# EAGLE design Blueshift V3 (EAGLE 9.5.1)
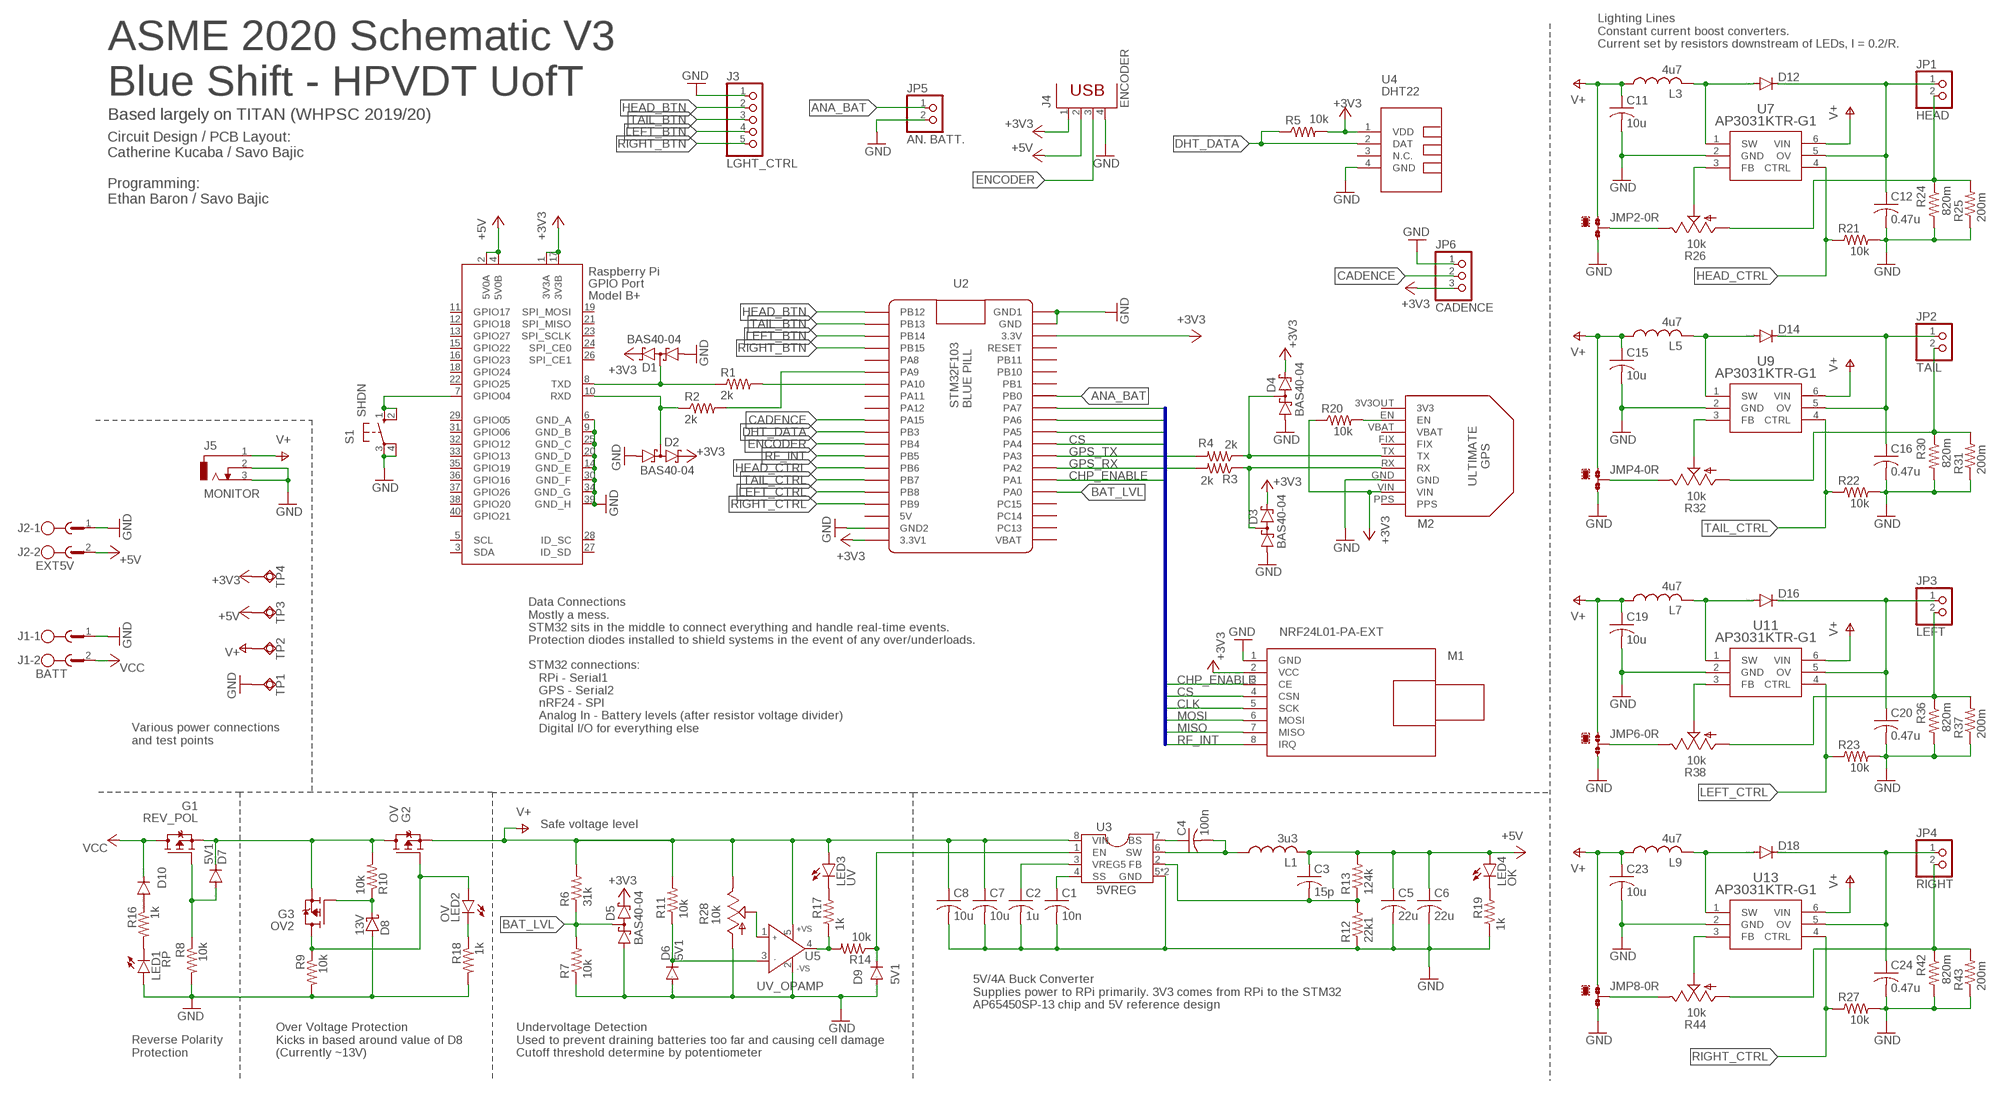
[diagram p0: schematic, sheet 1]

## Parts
C1  10n  C-USC0402  [C0402]
C2  1u  C-USC0402  [C0402]
C3  15p  C-USC0402  [C0402]
C4  100n  C-USC0402  [C0402]
C5  22u  C-USC0805  [C0805]
C6  22u  C-USC0805  [C0805]
C7  10u  C-USC0805  [C0805]
C8  10u  C-USC0805  [C0805]
C11  10u  C-USC1206K  [C1206K]
C12  0.47u  C-USC1206K  [C1206K]
C15  10u  C-USC1206K  [C1206K]
C16  0.47u  C-USC1206K  [C1206K]
C19  10u  C-USC1206K  [C1206K]
C20  0.47u  C-USC1206K  [C1206K]
C23  10u  C-USC1206K  [C1206K]
C24  0.47u  C-USC1206K  [C1206K]
D1  BAS40-04  [SOT23]
D2  BAS40-04  [SOT23]
D3  BAS40-04  [SOT23]
D4  BAS40-04  [SOT23]
D5  BAS40-04  [SOT23]
D6  5V1  DIODE-SOD323-R  [SOD323-R]
D7  5V1  DIODE-SOD323-R  [SOD323-R]
D8  13V  BAS70  [SOT23]
D9  5V1  DIODE-SOD323-R  [SOD323-R]
D10  DIODE-SOD80C  [SOD80C]
D12  DIODE-DO-214AC  [DO-214AC]
D14  DIODE-DO-214AC  [DO-214AC]
D16  DIODE-DO-214AC  [DO-214AC]
D18  DIODE-DO-214AC  [DO-214AC]
G1  REV_POL  SI3493DDV-T1-GE3  [TSOP-6]
G2  OV  SI3493DDV-T1-GE3  [TSOP-6]
G3  OV2  SI3493DDV-T1-GE3  [TSOP-6]
J1  BATT  MST2V  [MSTBV2]
J2  EXT5V  MST2V  [MSTBV2]
J3  LGHT_CTRL  PINHD-1X5  [1X05]
J4  ENCODER  PN87520  [PN87520]
J5  MONITOR  DCJ0303  [DCJ0303]
JMP2  0R-JUMPA  [A0R-JMP]
JMP4  0R-JUMPA  [A0R-JMP]
JMP6  0R-JUMPA  [A0R-JMP]
JMP8  0R-JUMPA  [A0R-JMP]
JP1  HEAD  PINHD-1X2  [1X02]
JP2  TAIL  PINHD-1X2  [1X02]
JP3  LEFT  PINHD-1X2  [1X02]
JP4  RIGHT  PINHD-1X2  [1X02]
JP5  AN. BATT.  PINHD-1X2  [1X02]
JP6  CADENCE  PINHD-1X3  [1X03]
L1  3u3  SDES064T-3R3MS  [SDES064T]
L3  4u7  NR6028NR6028  [INDDFN600X600X280-2N]
L5  4u7  NR6028NR6028  [INDDFN600X600X280-2N]
L7  4u7  NR6028NR6028  [INDDFN600X600X280-2N]
L9  4u7  NR6028NR6028  [INDDFN600X600X280-2N]
LED1  RP  LEDSML0805  [SML0805]
LED2  OV  LEDSML0805  [SML0805]
LED3  UV  LEDSML0805  [SML0805]
LED4  OK  LEDSML0805  [SML0805]
M1  NRF24L01-PA-EXT  WIRELESS-NRF24L01-PA-EXT  [WIRELESS-NRF24L01-PA-EXT]
M2  ULTIMATE-GPS  [ULTIMATE_GPS]
R1  2k  R-US_R0402  [R0402]
R2  2k  R-US_R0402  [R0402]
R3  2k  R-US_R0402  [R0402]
R4  2k  R-US_R0402  [R0402]
R5  10k  R-US_R0402  [R0402]
R6  31k  R-US_R0402  [R0402]
R7  10k  R-US_R0402  [R0402]
R8  10k  R-US_R0402  [R0402]
R9  10k  R-US_R0402  [R0402]
R10  10k  R-US_R0402  [R0402]
R11  10k  R-US_R0402  [R0402]
R12  22k1  R-US_R0402  [R0402]
R13  124k  R-US_R0402  [R0402]
R14  10k  R-US_R0402  [R0402]
R16  1k  R-US_R0402  [R0402]
R17  1k  R-US_R0402  [R0402]
R18  1k  R-US_R0402  [R0402]
R19  1k  R-US_R0402  [R0402]
R20  10k  R-US_R0402  [R0402]
R21  10k  R-US_R0402  [R0402]
R22  10k  R-US_R0402  [R0402]
R23  10k  R-US_R0402  [R0402]
R24  820m  R-US_R0603  [R0603]
R25  200m  R-US_R0805  [R0805]
R26  10k  TRIM_US-RJ9W  [RJ9W]
R27  10k  R-US_R0402  [R0402]
R28  10k  TRIM_US-RJ9W  [RJ9W]
R30  820m  R-US_R0603  [R0603]
R31  200m  R-US_R0805  [R0805]
R32  10k  TRIM_US-RJ9W  [RJ9W]
R36  820m  R-US_R0603  [R0603]
R37  200m  R-US_R0805  [R0805]
R38  10k  TRIM_US-RJ9W  [RJ9W]
R42  820m  R-US_R0603  [R0603]
R43  200m  R-US_R0805  [R0805]
R44  10k  TRIM_US-RJ9W  [RJ9W]
S1  SHDN  10-XX  [B3F-10XX]
TP1  TPSQTP20SQ  [TP20SQ]
TP2  TPSQTP20R  [TP20R]
TP3  TPSQTP20R  [TP20R]
TP4  TPSQTP20R  [TP20R]
U1  RASPI_HAT  [RASPI_BOARD_B+HAT_CF]
U2  BLUEPILL  BLUE_PILL  [BLUE_PILL]
U3  5VREG  AP65450SP-13  [SO-8EP]
U4  DHT22  TEMP-HUM-SENSOR-DHT22  [TEMP-HUM-SENSOR-DHT22]
U5  UV_OPAMP  TA75S558F,LF  [SOT-753]
U7  AP3031KTR-G1  [SOT23-6]
U9  AP3031KTR-G1  [SOT23-6]
U11  AP3031KTR-G1  [SOT23-6]
U13  AP3031KTR-G1  [SOT23-6]

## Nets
5V_FB: C3.2 R12.2 R13.1 U3.2(FB)
+3V3: D1.2(C2) D2.2(C2) D3.2(C2) D4.2(C2) D5.2(C2) J4.1 JP6.3 M1.2(VCC) M2.VIN R5.2 R20.1 TP4.TP U1.1(3V3A) U1.17(3V3B) U2.P$20(3.3V1) U2.P$23(3.3V) U4.1(VDD)
+5V: C3.1 C5.1 C6.1 J2.2 J4.2 L1.2 LED4.A R13.2 TP3.TP U1.2(5V0A) U1.4(5V0B)
ANA_BAT: JP5.1 U2.P$28(PB0)
BAT_LVL: D5.3(C1A2) R6.1 R7.2 U2.P$36(PA0)
CADENCE: JP6.2 U2.P$10(PA15)
CHP_ENABLE: M1.3(CE) U2.P$35(PA1)
CLK: M1.5(SCK) U2.P$31(PA5)
CS: M1.4(CSN) U2.P$32(PA4)
DHT_DATA: R5.1 U2.P$11(PB3) U4.2(DAT)
ENCODER: J4.3 U2.P$12(PB4)
GND: C1.2 C2.2 C5.2 C6.2 C7.2 C8.2 C11.2 C12.2 C15.2 C16.2 C19.2 C20.2 C23.2 C24.2 D1.1(A1) D2.1(A1) D3.1(A1) D4.1(A1) D5.1(A1) D6.A D8.1(A) D9.A J1.1 J2.1 J3.1 J4.4 J5.2 J5.3 JMP2.3 JMP4.3 JMP6.3 JMP8.3 JP5.2 JP6.1 LED1.A M1.1(GND) M2.GND R7.1 R8.2 R9.2 R12.1 R18.2 R19.1 R21.2 R22.2 R23.2 R24.2 R25.1 R27.2 R28.A R30.2 R31.1 R36.2 R37.1 R42.2 R43.1 S1.3(P) S1.4(P1) TP1.TP U1.6(GND_A) U1.9(GND_B) U1.14(GND_E) U1.20(GND_D) U1.25(GND_C) U1.30(GND_F) U1.34(GND_G) U1.39(GND_H) U2.P$19(GND2) U2.P$21(GND1) U2.P$22(GND) U3.5(GND) U3.TP(GND) U4.4(GND) U5.2(-VS) U7.2(GND) U9.2(GND) U11.2(GND) U13.2(GND)
GPS_RX: R3.2 U2.P$34(PA2)
GPS_TX: R4.2 U2.P$33(PA3)
HEAD_BTN: J3.2 U2.P$1(PB12)
HEAD_CTRL: R21.1 U2.P$14(PB6) U7.4(CTRL)
LEFT_BTN: J3.4 U2.P$3(PB14)
LEFT_CTRL: R23.1 U2.P$16(PB8) U11.4(CTRL)
MISO: M1.7(MISO) U2.P$30(PA6)
MOSI: M1.6(MOSI) U2.P$29(PA7)
N$1: R1.2 U2.P$7(PA10)
N$2: R2.2 U2.P$6(PA9)
N$3: D1.3(C1A2) R1.1 U1.8(TXD)
N$4: D2.3(C1A2) R2.1 U1.10(RXD)
N$5: D3.3(C1A2) M2.RX R3.1
N$6: S1.1(S) S1.2(S1) U1.7(GPIO04)
N$7: D8.3(C) G3.3(G) R10.1
N$8: D7.A G1.3(G) R8.1
N$9: D4.3(C1A2) M2.TX R4.1
N$10: G2.3(G) G3.1(D) G3.2(D) G3.5(D) G3.6(D) LED2.A R9.1
N$11: LED3.C R17.2
N$12: C1.1 U3.4(SS)
N$13: D6.C R11.1 U5.3(IN-)
N$14: C4.2 L1.1 U3.6(SW)
N$15: C2.1 U3.3(VREG5)
N$16: C4.1 U3.7(BS)
N$17: R14.2 R17.1 U5.4(OUT)
N$18: D9.C R14.1 U3.1(EN)
N$19: R28.S U5.1(IN+)
N$20: LED1.C R16.2
N$21: D10.A R16.1
N$22: M2.EN R20.2
N$23: LED2.C R18.1
N$24: LED4.C R19.2
N$25: D7.C G1.4(S) G2.1(D) G2.2(D) G2.5(D) G2.6(D) G3.4(S) R10.2
N$31: D12.A L3.2 U7.1(SW)
N$32: JMP2.2 R26.E
N$33: R26.S U7.3(FB)
N$34: C12.1 D12.C JP1.1 U7.5(OV)
N$35: JP1.2 R24.1 R25.2 R26.A
N$41: D14.A L5.2 U9.1(SW)
N$42: JMP4.2 R32.E
N$43: R32.S U9.3(FB)
N$44: C16.1 D14.C JP2.1 U9.5(OV)
N$45: JP2.2 R30.1 R31.2 R32.A
N$51: D16.A L7.2 U11.1(SW)
N$52: JMP6.2 R38.E
N$53: R38.S U11.3(FB)
N$54: C20.1 D16.C JP3.1 U11.5(OV)
N$55: JP3.2 R36.1 R37.2 R38.A
N$61: D18.A L9.2 U13.1(SW)
N$62: JMP8.2 R44.E
N$63: R44.S U13.3(FB)
N$64: C24.1 D18.C JP4.1 U13.5(OV)
N$65: JP4.2 R42.1 R43.2 R44.A
RF_INT: M1.8(IRQ) U2.P$13(PB5)
RIGHT_BTN: J3.5 U2.P$4(PB15)
RIGHT_CTRL: R27.1 U2.P$17(PB9) U13.4(CTRL)
TAIL_BTN: J3.3 U2.P$2(PB13)
TAIL_CTRL: R22.1 U2.P$15(PB7) U9.4(CTRL)
V+: C7.1 C8.1 C11.1 C15.1 C19.1 C23.1 G2.4(S) J5.1 JMP2.1 JMP4.1 JMP6.1 JMP8.1 L3.1 L5.1 L7.1 L9.1 LED3.A R6.2 R11.2 R28.E TP2.TP U3.8(VIN) U5.5(+VS) U7.6(VIN) U9.6(VIN) U11.6(VIN) U13.6(VIN)
VCC: D10.C G1.1(D) G1.2(D) G1.5(D) G1.6(D) J1.2
Unconnected: M2.3V3OUT(3V3) M2.FIX M2.PPS M2.VBAT U1.3(SDA) U1.5(SCL) U1.11(GPIO17) U1.12(GPIO18) U1.13(GPIO27) U1.15(GPIO22) U1.16(GPIO23) U1.18(GPIO24) U1.19(SPI_MOSI) U1.21(SPI_MISO) U1.22(GPIO25) U1.23(SPI_SCLK) U1.24(SPI_CE0) U1.26(SPI_CE1) U1.27(ID_SD) U1.28(ID_SC) U1.29(GPIO05) U1.31(GPIO06) U1.32(GPIO12) U1.33(GPIO13) U1.35(GPIO19) U1.36(GPIO16) U1.37(GPIO26) U1.38(GPIO20) U1.40(GPIO21) U2.P$5(PA8) U2.P$8(PA11) U2.P$9(PA12) U2.P$18(5V) U2.P$24(RESET) U2.P$25(PB11) U2.P$26(PB10) U2.P$27(PB1) U2.P$37(PC15) U2.P$38(PC14) U2.P$39(PC13) U2.P$40(VBAT) U4.3(N.C.)

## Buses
SPI:CHP_ENABLE,CLK,CS,MISO,MOSI,RF_INT

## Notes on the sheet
- Lighting Lines
  Constant current boost converters. 
  Current set by resistors downstream of LEDs, I = 0.2/R.
- ASME 2020 Schematic V3
  Blue Shift - HPVDT UofT
- Based largely on TITAN (WHPSC 2019/20)
- Circuit Design / PCB Layout:
  Catherine Kucaba / Savo Bajic
  
  Programming:
  Ethan Baron / Savo Bajic
- Data Connections
  Mostly a mess.
  STM32 sits in the middle to connect everything and handle real-time events.
  Protection diodes installed to shield systems in the event of any over/underloads.
  
  STM32 connections:
     RPi - Serial1
     GPS - Serial2
     nRF24 - SPI
     Analog In - Battery levels (after resistor voltage divider)
     Digital I/O for everything else
- Various power connections
  and test points
- Safe voltage level
- 5V/4A Buck Converter
  Supplies power to RPi primarily. 3V3 comes from RPi to the STM32
  AP65450SP-13 chip and 5V reference design
- Reverse Polarity
  Protection
- Over Voltage Protection
  Kicks in based around value of D8
  (Currently ~13V)
- Undervoltage Detection
  Used to prevent draining batteries too far and causing cell damage
  Cutoff threshold determine by potentiometer

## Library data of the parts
C1-C8 C11 C12 C15 C16 C19 C20 C23 C24 = rcl:C-US: CAPACITOR, American symbol; SPICEPREFIX: C
D1-D5 = diode:BAS40-04: Silicon Schottky Diodes General-purpose diode for high-speed switching
D6 D7 D9 D10 D12 D14 D16 D18 = diode:DIODE-: DIODE
D8 = diode:BAS70: Silicon Schottky Diodes
G1-G3 = ASME2020_parts:SI3493DDV-T1-GE3: 20V P-CH MOSFET
J1 J2 = con-phoenix-508:MST2V: PHOENIX; OC_FARNELL: unknown; OC_NEWARK: unknown
J3 = pinhead:PINHD-1X5: PIN HEADER
J4 = con-berg:PN87520: BERG USB connector; OC_FARNELL: unknown; OC_NEWARK: unknown
J5 = con-jack:DCJ0303: DC POWER JACK Source: DCJ0303.pdf; OC_FARNELL: unknown; OC_NEWARK: unknown
JMP2 JMP4 JMP6 JMP8 = jump-0r-smd:0R-JUMP: SMD 0R 0805 Jumper
JP1-JP5 = pinhead:PINHD-1X2: PIN HEADER
JP6 = pinhead:PINHD-1X3: PIN HEADER
L1 = ASME2020_parts:SDES064T-3R3MS
L3 L5 L7 L9 = Lighting IC:NR6028
LED1-LED4 = led:LED: LED
M1 = diy-modules:WIRELESS-NRF24L01-PA-EXT: 2.4 GHz Wireless Module based on NRF24L01 chip with preamplifier and external antenna Click here to find device on ebay.com
M2 = diy-modules:ULTIMATE-GPS
R1-R14 R16-R25 R27 R30 R31 R36 R37 R42 R43 = rcl:R-US_: RESISTOR, American symbol; SPICEPREFIX: R
R26 R28 R32 R38 R44 = pot:TRIM_US-: POTENTIOMETER
S1 = switch-omron:10-XX: OMRON SWITCH; MPN: B3F-1000; OC_FARNELL: 176432; OC_NEWARK: 36M3542
TP1-TP4 = testpad:TPSQ: Test pad
U1 = raspberrypi_bastelstube_v13:RASPI_HAT
U2 = BluePill:BLUE_PILL
U3 = ASME2020_parts:AP65450SP-13: AP65450 4A, 18V, 650kHz ADAPTIVE COT STEP-DOWN CONVERTER
U4 = diy-modules:TEMP-HUM-SENSOR-DHT22: DHT22 - digital humidity & temperature sensor Also known as: AM2302 AM2302 datasheet available here: http://akizukidenshi.com/download/ds/aosong/AM2302.pdf Click here to find device on ebay.com
U5 = ASME2020_parts:TA75S558F,LF
U7 U9 U11 U13 = Lighting IC:AP3031KTR-G1: AP3031 step-up LED driver chip for LEDs up to 1.4A; MANUFACTURER_PART_NUMBER: AP3031KTRG1; VENDOR: Diodes Inc

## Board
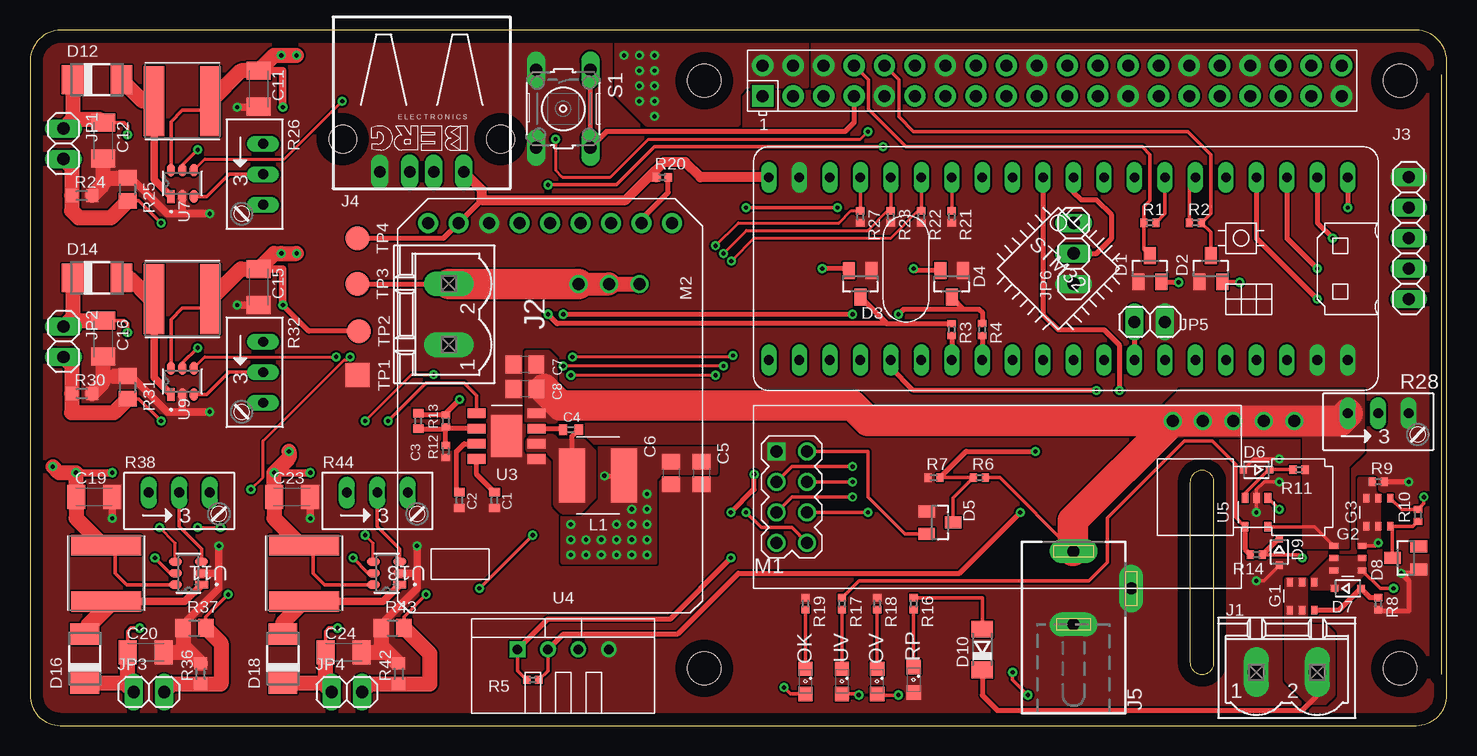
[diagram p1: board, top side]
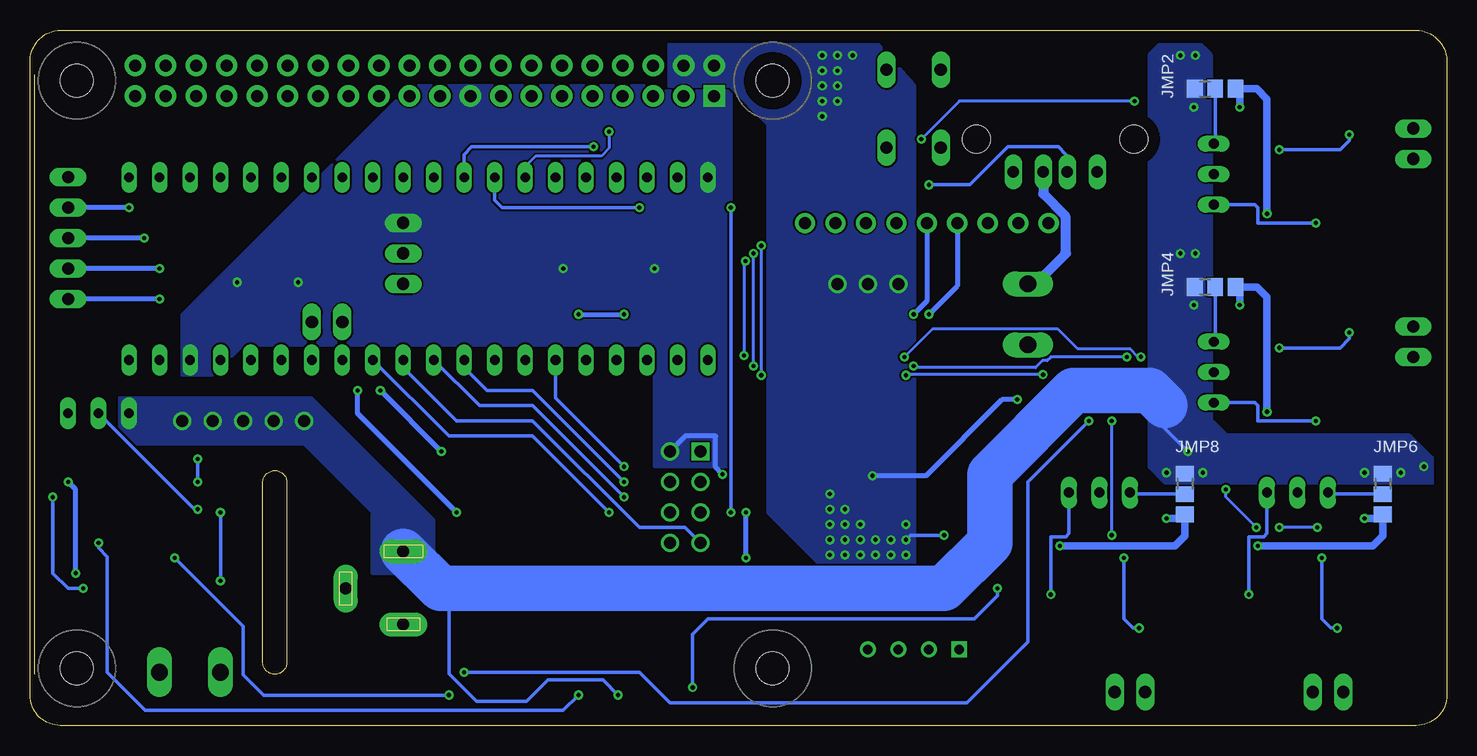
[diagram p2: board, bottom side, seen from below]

Size 118.11 x 58 mm. Coordinates in mm from the lower left corner, seen from the top.
Outline: 2.54,0 115.57,0 arc90 118.11,2.54 118.11,55.24 arc90 115.57,58 2.54,58 arc90 0,55.24 0,2.54 arc90 2.54,0
Copper layers (1*16): Top 0.035mm / dielectric 1.5mm / Bottom 0.035mm
Design rules "default": minimum track width 6mil, minimum drill 0.35mm, track to track 6mil, track to pad 6mil, pad to pad 6mil, via to via 6mil, smd to smd 6mil, copper to edge 40mil, drill to drill 6mil, minimum pad ring 10mil, minimum via ring 8mil, stop-mask expansion 4mil, vias tented up to drill 0mil, thermal gap 10mil

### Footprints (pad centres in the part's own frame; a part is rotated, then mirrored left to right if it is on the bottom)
C0402 = smd 0.7 x 0.9: 1 -0.65,0; 2 0.65,0
C0805 = smd 1.3 x 1.5: 1 -0.95,0; 2 0.95,0
C1206K = smd 1.5 x 2: 1 -1.5,0; 2 1.5,0
SOT23 = smd 1 x 1.4: 1 -0.95,-1.1; 2 0.95,-1.1; 3 0,1.1
SOD323-R = smd 0.6 x 0.6: A 1.1,0; C -1.1,0
SOD80C = smd 1.4 x 1.8: A 1.7,0; C -1.7,0
DO-214AC = smd 1.8 x 2.4: A 2.025,0; C -2.025,0
TSOP-6 = smd 0.508 x 0.711: 1 -1.016,-1.168; 2 0,-1.168; 3 1.016,-1.168; 4 1.016,1.168; 5 0,1.168; 6 -1.016,1.168
MSTBV2 = drill 1.397 long: 1 -2.54,0; 2 2.54,0
1X05 = drill 1.016 long: 1 -5.08,0; 2 -2.54,0; 3 0,0; 4 2.54,0; 5 5.08,0
PN87520 = drill 0.95 long: 1 -3.5,2.71; 2 -1,2.71; 3 1,2.71; 4 3.5,2.71 | hole 2.3: -6.57,0; 6.57,0
DCJ0303 = drill 1 pad 2 long: 1 0,3.1; 2 4.8,0; 3 0,-3
A0R-JMP = smd 1.5 x 1.3: 1 0,1.7; 2 0,0; 3 0,-1.7
1X02 = drill 1.016 long: 1 -1.27,0; 2 1.27,0
1X03 = drill 1.016 long: 1 -2.54,0; 2 0,0; 3 2.54,0
SDES064T = smd 2.15 x 4.5: 1 -2.175,0; 2 2.175,0
INDDFN600X600X280-2N = smd 1.712 x 5.812: 1 -2.35,0; 2 2.35,0
SML0805 = smd 1.2 x 1.2: A 1.05,0; C -1.05,0
WIRELESS-NRF24L01-PA-EXT = drill 1 square: 1 -18.415,3.81 | drill 1: 2 -15.875,3.81; 3 -18.415,1.27; 4 -15.875,1.27; 5 -18.415,-1.27; 6 -15.875,-1.27; 7 -18.415,-3.81; 8 -15.875,-3.81
ULTIMATE_GPS = drill 1 pad 1.676: 3V3OUT 0,10.16; EN 0,7.62; FIX 0,2.54; GND 0,-5.08; PPS 0,-10.16; RX 0,-2.54; TX 0,0; VBAT 0,5.08; VIN 0,-7.62
R0402 = smd 0.6 x 0.7: 1 -0.5,0; 2 0.5,0
R0603 = smd 1 x 1.1: 1 -0.85,0; 2 0.85,0
R0805 = smd 1.3 x 1.5: 1 -0.95,0; 2 0.95,0
RJ9W = drill 0.813 long: A 2.54,0.635; E -2.54,0.635; S 0,0.635
B3F-10XX = drill 1.016 long: 1 -3.251,2.261; 2 3.251,2.261; 3 -3.251,-2.261; 4 3.251,-2.261
TP20SQ = smd 2 x 2: TP 0,0
TP20R = smd 2 x 2: TP 0,0
RASPI_BOARD_B+HAT_CF = drill 1 pad 1.778 square: 1 8.37,51.23 | drill 1 pad 1.778: 2 8.37,53.77; 3 10.91,51.23; 4 10.91,53.77; 5 13.45,51.23; 6 13.45,53.77; 7 15.99,51.23; 8 15.99,53.77; 9 18.53,51.23; 10 18.53,53.77; 11 21.07,51.23; 12 21.07,53.77; 13 23.61,51.23; 14 23.61,53.77; 15 26.15,51.23; 16 26.15,53.77; 17 28.69,51.23; 18 28.69,53.77; 19 31.23,51.23; 20 31.23,53.77; 21 33.77,51.23; 22 33.77,53.77; 23 36.31,51.23; 24 36.31,53.77; 25 38.85,51.23; 26 38.85,53.77; 27 41.39,51.23; 28 41.39,53.77; 29 43.93,51.23; 30 43.93,53.77; 31 46.47,51.23; 32 46.47,53.77; 33 49.01,51.23; 34 49.01,53.77; 35 51.55,51.23; 36 51.55,53.77; 37 54.09,51.23; 38 54.09,53.77; 39 56.63,51.23; 40 56.63,53.77 | hole 2.75: 3.5,3.5; 3.5,52.5; 61.5,3.5; 61.5,52.5
BLUE_PILL = drill 0.8 long: P$1 -7.62,15.24; P$2 -7.62,12.7; P$3 -7.62,10.16; P$4 -7.62,7.62; P$5 -7.62,5.08; P$6 -7.62,2.54; P$7 -7.62,0; P$8 -7.62,-2.54; P$9 -7.62,-5.08; P$10 -7.62,-7.62; P$11 -7.62,-10.16; P$12 -7.62,-12.7; P$13 -7.62,-15.24; P$14 -7.62,-17.78; P$15 -7.62,-20.32; P$16 -7.62,-22.86; P$17 -7.62,-25.4; P$18 -7.62,-27.94; P$19 -7.62,-30.48; P$20 -7.62,-33.02; P$21 7.62,15.24; P$22 7.62,12.7; P$23 7.62,10.16; P$24 7.62,7.62; P$25 7.62,5.08; P$26 7.62,2.54; P$27 7.62,0; P$28 7.62,-2.54; P$29 7.62,-5.08; P$30 7.62,-7.62; P$31 7.62,-10.16; P$32 7.62,-12.7; P$33 7.62,-15.24; P$34 7.62,-17.78; P$35 7.62,-20.32; P$36 7.62,-22.86; P$37 7.62,-25.4; P$38 7.62,-27.94; P$39 7.62,-30.48; P$40 7.62,-33.02
SO-8EP = smd 0.802 x 1.505: 1 -1.905,-2.498; 2 -0.635,-2.498; 3 0.635,-2.498; 4 1.905,-2.498; 5 1.905,2.498; 6 0.635,2.498; 7 -0.635,2.498; 8 -1.905,2.498 | smd 3.502 x 2.613: TP 0,0
TEMP-HUM-SENSOR-DHT22 = drill 0.8 square: 1 -3.81,0 | drill 0.8: 2 -1.27,0; 3 1.27,0; 4 3.81,0
SOT-753 = smd 0.8 x 0.55: 1 -1.2,0.95; 2 -1.2,0; 3 -1.2,-0.95; 4 1.2,-0.95; 5 1.2,0.95
SOT23-6 = smd 1.06 x 0.65: 1 -1.1,0.95; 2 -1.1,0; 3 -1.1,-0.95; 4 1.1,-0.95; 5 1.1,0; 6 1.1,0.95

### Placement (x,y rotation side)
C1  38.72,18.8 270 top
C2  35.8,18.8 270 top
C3  32.37,25.4 270 top
C4  45.08,24.67 0 top
C5  55.98,21.06 270 top
C6  53.44,21.06 270 top
C7  41.26,30.1 180 top
C8  41.26,28.07 180 top
C11  19.05,53.09 270 top
C12  6.1,48.77 270 top
C15  19.05,36.58 270 top
C16  6.1,32.26 270 top
C19  5.33,19.05 0 top
C20  9.65,6.1 0 top
C23  21.84,19.05 0 top
C24  26.16,6.1 0 top
D1  93.34,38.1 0 top
D2  98.42,38.1 0 top
D3  69.22,36.83 180 top
D4  76.84,36.83 180 top
D5  75.85,16.93 270 top
D6  102.23,21.32 180 top
D7  109.86,11.43 0 top
D8  114.68,13.97 90 top
D9  104.14,14.48 270 top
D10  79.38,6.35 90 top
D12  5.59,53.85 0 top
D14  5.59,37.34 0 top
D16  4.57,5.59 90 top
D18  21.08,5.59 90 top
G1  106.05,10.79 0 top
G2  109.86,13.97 90 top
G3  112.39,17.78 0 top
J1  104.78,4.45 0 top
J2  34.92,34.29 90 top
J3  114.94,40.64 270 top
J4  32.65,48.89 180 top
J5  87,11.43 0 top
JMP2  19.3,53.09 90 bottom
JMP4  19.3,36.58 90 bottom
JMP6  5.33,19.3 0 bottom
JMP8  21.84,19.3 0 bottom
JP1  2.79,48.51 270 top
JP2  2.79,32 270 top
JP3  9.91,2.79 0 top
JP4  26.42,2.79 0 top
JP5  93.34,33.66 0 top
JP6  87,39.37 90 top
L1  47.36,20.86 0 top
L3  12.7,52.07 180 top
L5  12.7,35.56 180 top
L7  6.35,12.7 270 top
L9  22.86,12.7 270 top
LED1  73.66,3.81 270 top
LED2  70.61,3.68 270 top
LED3  67.69,3.68 270 top
LED4  64.64,3.68 270 top
M1  80.64,19.05 0 top
M2  43.36,41.91 270 top
R1  93.34,41.91 0 top
R2  97.16,41.91 180 top
R3  76.84,33.02 270 top
R4  79.38,33.02 270 top
R5  41.91,3.81 180 top
R6  79.16,20.67 0 top
R7  75.34,20.67 0 top
R8  112.39,10.16 270 top
R9  112.39,20.32 0 top
R10  115.7,17.53 90 top
R11  105.79,21.34 0 top
R12  34.66,22.86 90 top
R13  34.66,25.4 90 top
R14  102.23,14.24 180 top
R16  73.66,10.16 270 top
R17  67.69,10.16 270 top
R18  70.61,10.16 90 top
R19  64.64,10.16 270 top
R20  52.7,45.72 0 top
R21  76.84,42.42 270 top
R22  74.3,42.42 270 top
R23  71.75,42.42 270 top
R24  4.32,44.2 0 top
R25  8.13,44.7 270 top
R26  18.8,45.97 270 top
R27  69.22,42.42 270 top
R28  112.39,25.4 0 top
R30  4.32,27.69 0 top
R31  8.13,28.19 270 top
R32  18.8,29.46 270 top
R36  14.22,4.32 90 top
R37  13.72,8.13 0 top
R38  12.45,18.8 0 top
R42  30.73,4.32 90 top
R43  30.23,8.13 0 top
R44  28.96,18.8 0 top
S1  44.45,51.44 270 top
TP1  27.3,29.21 270 top
TP2  27.43,32.89 270 top
TP3  27.3,36.83 270 top
TP4  27.3,40.64 270 top
U1  52.7,1.27 0 top
U2  94.61,38.1 270 top
U3  39.73,24.13 270 top
U4  44.45,6.35 0 top
U5  102.23,17.78 270 top
U7  12.7,45.21 90 top
U9  12.7,28.7 90 top
U11  13.21,12.7 180 top
U13  29.72,12.7 180 top

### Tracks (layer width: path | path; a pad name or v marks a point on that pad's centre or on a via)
5V_FB
  Top 0.406: R12.2 R13.1 | U3.2 34.79,24.77 R13.1 | C3.2 34.5,24.75 R13.1
+3V3  (via drill 0.35)
  Top 0.305: D5.2 72.92,15.97 69.85,19.05 69.85,22.86 M1.2 | R5.2 40.64,4.58 U4.1
  Top 0.406: 37.64,43.81 M2.VIN 34.47,40.64 TP4.TP | D3.2 68.09,38.1 v66.04,38.1 | D4.2 73.83,37.93 v73.66,38.1 | D1.2 95.72,37 v95.76,36.96 | D2.2 100.8,37 v100.84,36.96 | U4.1 43.18,8.89 53.39,8.89 55.88,11.38 55.88,11.43 v58.42,13.97 | v60.37,20.95 60.37,19.68 60.33,19.68 v58.42,17.78
  Top 0.813: J4.1 37.64,44.69 37.64,43.81 49.67,43.81 51.57,45.72 | R20.1 51.57,45.72 | U2.P$20 55.88,45.72 54.61,46.99 52.84,46.99 51.57,45.72
  Bottom 0.406: v58.42,13.97 v58.42,17.78 | v60.37,20.95 60.96,21.54 60.96,24.13 63.5,24.13 M1.2
  pour Bottom (rank 2, no thermals): 59.69,21.59 59.69,53.34 86.36,53.34 105.41,34.29 105.41,29.21 102.87,29.21 100.33,31.75 66.04,31.75 66.04,21.59
+5V  (via drill 0.35, 1)
  Top 0.305: LED4.A 63.41,2.63 v62.87,3.17 | v37.47,11.43 v41.91,15.88
  Top 0.406: C3.1 32.52,25.9 R13.2 34.66,26.02 v35.81,27.18 | v47.88,20.83 49.5,20.83 L1.2 | TP3.TP J2.2
  Top 1.27: v48.26,36.83 v50.8,36.83
  Top 1.905: v45.72,36.83 v48.26,36.83
  Top 2.54: J2.2 v45.72,36.83
  Bottom 0.305: v62.87,3.17 62.87,7.62 61.59,8.89 39.37,8.89 37.47,10.79 v37.47,11.43 | v41.91,15.88 44.7,15.88 v45.08,15.49
  Bottom 0.406: v35.81,27.18 37.08,27.18 43.43,20.83 v47.88,20.83
  Bottom 0.813: J4.2 33.65,44.34 31.8,42.49 31.8,39.42 31.75,39.37 34.29,36.83 J2.2
  other vias: 49.53,55.88 50.8,55.88 52.07,55.88 50.8,54.61 52.07,54.61 50.8,53.34 52.07,53.34 50.8,52.07 52.07,52.07 52.07,50.8 51.44,19.3 51.44,18.03 50.17,18.03 50.17,16.76 48.89,16.76 51.44,16.76 51.44,15.49 50.17,15.49 48.89,15.49 47.62,15.49 46.36,15.49 45.08,16.76 45.08,14.22 46.36,14.22 47.62,14.22 48.89,14.22 50.17,14.22 51.44,14.22
  pour Top (rank 2, no thermals): 44.45,13.59 44.45,23.11 57.15,23.11 57.15,21.08 52.58,21.08 52.07,20.57 52.07,13.59
  pour Bottom (no thermals): 44.45,53.34 44.45,13.34 52.07,13.34 56.52,17.78 56.52,50.16 59.69,53.34 64.77,53.34 64.77,57.78 48.36,57.78
  pour Top (no thermals): 48.89,57.78 48.89,52.7 51.44,50.16 59.05,50.16 59.05,52.7 59.69,53.34 64.77,53.34 64.77,57.78
ANA_BAT
  Top 0.406: JP5.1 U2.P$28
BAT_LVL  (via drill 0.35)
  Top 0.305: D5.3 76.95,18.96 R6.1 R7.2
  Top 0.406: R7.2 78.03,22.86 v83.82,22.86 | v88.9,27.94 73.66,27.94 71.75,29.84 U2.P$36
  Bottom 0.406: v83.82,22.86 v88.9,27.94
CADENCE
  Top 0.406: JP6.2 88.9,39.37 90.17,40.64 90.17,42.55 88.9,43.81 87.63,43.81 87,44.45 U2.P$10
CHP_ENABLE  (via drill 0.35)
  Top 0.305: M1.3 63.5,21.59 v68.58,21.59
  Bottom 0.305: U2.P$35 74.3,27.3 v68.58,21.59
CLK  (via drill 0.35)
  Top 0.305: M1.5 63.5,19.05 v68.58,19.05
  Bottom 0.305: U2.P$31 80.64,26.67 76.2,26.67 v68.58,19.05
CS  (via drill 0.35)
  Top 0.305: M1.4 v68.58,20.32
  Bottom 0.305: U2.P$32 81.91,29.84 80.01,27.94 76.2,27.94 v68.58,20.32
DHT_DATA  (via drill 0.35)
  Top 0.305: R5.1 43.18,4.58 U4.2
  Top 0.406: U4.2 44.45,7.62 53.97,7.62 59.05,12.7 77.47,12.7 v82.55,17.78 | v90.81,27.94 90.81,31.75 89.53,33.02 85.72,33.02 84.45,34.29 U2.P$11
  Bottom 0.406: v90.81,27.94 90.81,26.04 v82.55,17.78
ENCODER  (via drill 0.35)
  Top 0.305: v43.18,45.09 48.89,45.09 52.07,48.26 v71.12,48.26
  Bottom 0.305: J4.3 31.75,46.28 31.75,47.62 32.39,48.26 36.57,48.26 39.75,45.09 v43.18,45.09 | v71.12,48.26 81.28,48.26 81.91,47.62 U2.P$12
GND  (via drill 0.35)
  Top 0.305: D6.A 102.04,22.23 v104.14,22.23 | v104.14,20.32 102.88,20.32 102.23,19.67 U5.2 v102.23,17.78 | v102.23,12.06 102.87,12.06 104.14,13.34 D9.A
  Top 0.406: D8.1 115.46,12.7 v114.3,12.7 114.94,12.06 114.94,9.53 112.53,9.53 R8.2 | v114.94,20.32 R9.2
  Top 0.635: 12.7,42.67 11.43,42.67 8.45,45.65 R25.1 | 12.7,42.67 U7.2 | v14.99,42.67 12.7,42.67 | v17.27,51.56 19.03,51.56 C11.2 | 6.1,45.12 6.1,45.97 C12.2 | 12.7,26.16 11.43,26.16 8.45,29.14 R31.1 | 12.7,26.16 U9.2 | v14.99,26.16 12.7,26.16 | v17.27,35.05 19.03,35.05 C15.2 | 6.1,28.61 6.1,29.46 | 6.1,29.46 C16.2 | 6.1,29.46 6.42,29.14 6.98,29.14 | 15.75,12.7 15.75,11.43 12.77,8.45 R37.1 12.77,7.62 | 15.75,12.7 U11.2 | v15.75,14.99 15.75,12.7 | v6.86,17.27 6.86,19.03 C19.2 | 32.26,12.7 32.26,11.43 29.28,8.45 R43.1 29.28,6.42 28.96,6.1 | 32.26,12.7 U13.2 | v32.26,14.99 32.26,12.7 | v23.37,17.27 23.37,19.03 C23.2 | R42.2 29.81,6.1 28.96,6.1 | 28.96,6.1 C24.2
  Top 1.27: R30.2 6.1,28.61 C16.2 | 6.98,29.14 R31.1 | R24.2 6.1,45.12 C12.2 | 6.1,45.97 6.42,45.65 R25.1 | C24.2 29.81,6.1 | 29.81,6.1 30.6,5.3 | 30.6,5.3 30.65,5.3 | 30.6,5.3 30.56,5.3 30.49,5.24 | C20.2 13.3,6.1 | 13.3,6.1 R36.2 | R37.1 12.77,6.63 13.3,6.1 | R43.1 29.28,6.63 29.81,6.1
  Bottom 0.305: v104.14,22.23 v104.14,20.32 | v102.23,17.78 v102.23,12.06
  Bottom 0.406: v114.3,12.7 114.3,19.68 v114.94,20.32
  Bottom 0.635: v17.27,51.56 17.27,52.75 JMP2.3 15.83,53.09 14.99,52.25 v14.99,42.67 | v17.27,35.05 17.27,36.24 JMP4.3 15.83,36.58 14.99,35.74 v14.99,26.16 | v6.86,17.27 5.67,17.27 JMP6.3 5.33,15.83 6.17,14.99 v15.75,14.99 | v23.37,17.27 22.18,17.27 JMP8.3 21.84,15.83 22.68,14.99 v32.26,14.99
  pour Top (rank 6, no thermals): 0.27,57.78 118.11,57.78 118.11,0 0.27,0
GPS_RX
  Top 0.406: R3.2 U2.P$34
GPS_TX
  Top 0.406: R4.2 U2.P$33
HEAD_BTN  (via drill 0.35)
  Top 0.406: U2.P$1 v109.86,43.18
  Bottom 0.406: v109.86,43.18 J3.2
HEAD_CTRL  (via drill 0.35)
  Top 0.254: U7.4 14.58,47.24 21.19,47.24 25.13,51.18 25.15,51.18 v26.03,52.07 | v69.85,49.53 69.22,48.9 51.56,48.9 48.41,45.74 44.37,45.74 43.81,46.3 v43.81,48.9
  Top 0.305: U2.P$14 R21.1
  Bottom 0.254: v26.03,52.07 40.64,52.07 v43.81,48.9 | U2.P$14 76.84,46.61 75.95,47.5 70.48,47.5 69.85,48.13 v69.85,49.53
LEFT_BTN  (via drill 0.35)
  Top 0.406: v107.31,38.1 104.78,40.64 U2.P$3
  Bottom 0.406: v107.31,38.1 J3.4
LEFT_CTRL  (via drill 0.35)
  Top 0.254: U11.4 12.11,15.2 v10.8,16.51 | v13.97,16.51 v15.88,16.51 | v18.42,19.68 19.43,20.7 19.43,23.73 26.19,30.49 26.42,30.49 v26.67,30.74 | v57.81,29.97 v44.45,29.97 | v57.81,39.37 59.71,41.27 69.85,41.27 71.49,42.92 R23.1
  Top 0.305: U2.P$16 R23.1
  Bottom 0.254: v10.8,16.51 v13.97,16.51 | v15.88,16.51 18.42,19.05 v18.42,19.68 | v26.67,30.74 33.01,30.74 33.33,30.42 33.71,30.42 34.29,29.84 44.32,29.84 v44.45,29.97 | v57.81,29.97 v57.81,39.37
MISO
  Bottom 0.305: M1.7 63.5,16.51 67.31,16.51 76.2,25.4 82.55,25.4 87,29.84 U2.P$30
MOSI  (via drill 0.35)
  Top 0.305: M1.6 v69.85,17.78
  Bottom 0.305: v69.85,17.78 76.2,24.13 83.19,24.13 U2.P$29
N$1
  Top 0.305: R1.2 94.61,42.68 U2.P$7
N$2
  Top 0.305: R2.2 96.66,45.22 U2.P$6
N$3
  Top 0.305: U1.8 69.89,53.85 69.89,51.4 73.03,48.26 92.71,48.26 93.34,47.62 93.34,43.76 92.84,43.26 R1.1 92.84,39.7 D1.3
N$4
  Top 0.305: U1.10 72.43,53.85 72.43,50.76 73.66,49.53 96.52,49.53 98.42,47.62 98.42,42.68 R2.1 98.42,41.14 D2.3
N$5  (via drill 0.35)
  Top 0.406: D3.3 71.42,33.52 | 71.42,33.52 R3.1 | v43.18,34.29 43.95,33.52 71.42,33.52
  Bottom 0.406: M2.RX 40.81,36.66 v43.18,34.29
N$6
  Top 0.406: U1.7 68.69,50.28 67.94,49.53 48.06,49.53 S1.2 S1.1
N$7
  Top 0.305: D8.3 113.58,16.44 G3.3 115.28,16.61 R10.1
N$8
  Top 0.406: G1.3 109.15,9.63 D7.A 111.72,10.66 R8.1
N$9  (via drill 0.35)
  Top 0.406: 77.87,34.69 D4.3 | R4.1 79.38,34.46 79.14,34.69 77.87,34.69 | 77.87,34.69 72.79,34.69 v72.39,34.29 | v68.58,34.29 v44.45,34.29
  Bottom 0.406: v72.39,34.29 v68.58,34.29 | v44.45,34.29 43.36,35.38 M2.TX
N$10  (via drill 0.35)
  Top 0.305: LED2.A 70.7,2.54 v72.39,2.54 | v112.39,15.24 112.14,14.99 G2.3
  Bottom 0.305: v112.39,15.24 112.39,14.81 111.66,14.08 111.66,4.45 108.49,1.27 73.66,1.27 v72.39,2.54
  pour Top (no thermals): 112.39,19.05 112.39,15.24 112.14,14.99 110.87,14.99 110.87,20.57 111.89,20.57 112.01,20.45 112.01,19.43
N$11
  Top 0.305: R17.2 LED3.C
N$12
  Top 0.406: C1.1 37.24,20.93 U3.4
N$13
  Top 0.305: U5.3 101.28,19.37 103.23,21.32 D6.C 103.35,21.34 R11.1
N$14
  Top 0.406: L1.1 45.18,24.11 C4.2
  pour Top (no thermals): 41.91,24.13 43.56,24.13 43.94,23.75 46.1,23.75 46.99,22.86 46.99,19.05 45.72,17.78 44.45,17.78 43.81,18.41 43.81,22.23 43.18,22.86 41.66,22.86 41.53,22.99 41.53,23.75
N$15
  Top 0.406: C2.1 35.56,19.68 35.56,22.86 36.19,23.5 U3.3
N$16
  Top 0.406: U3.7 44.34,24.77 C4.1
N$17
  Top 0.305: R17.1 69.1,12.06 88.27,12.06 89.82,13.62 89.82,17.31 96.22,23.71 98.55,23.71 100.51,21.75 100.51,17.36 U5.4
  Top 0.406: U5.4 101.28,14.69 R14.2
N$18  (via drill 0.35)
  Top 0.305: R14.1 105.78,14.24 v106.05,13.97 | v83.19,2.54 81.91,3.81 v81.91,4.45 | U3.1 37.24,27.53 36.19,28.57 33.02,28.57 v29.84,25.4
  Top 0.406: R14.1 104.07,15.58 D9.C
  Bottom 0.305: v106.05,13.97 100.33,8.26 100.33,4.24 98.63,2.54 v83.19,2.54 | v81.91,4.45 67.31,4.45 64.77,1.91 40,1.91 34.92,6.99 34.92,20.32 v29.84,25.4
N$19  (via drill 0.35)
  Top 0.305: U5.1 103.19,18.98 v104.14,18.03
  Bottom 0.305: R28.S 104.39,18.03 v104.14,18.03
N$20
  Top 0.305: R16.2 LED1.C
N$21
  Top 0.305: D10.A 79.38,10.66 R16.1
N$22
  Top 0.406: M2.EN 50.97,42.22 53.2,44.45 R20.2
N$23
  Top 0.305: LED2.C R18.1
N$24
  Top 0.305: R19.2 LED4.C
N$25  (via drill 0.35)
  Top 0.305: G3.4 114.33,18.03 R10.2 116.2,18.53 v116.2,19.05 | G2.1 112.55,11.43 v113.66,11.43
  Bottom 0.305: v113.66,11.43 114.94,11.43 116.2,12.7 v116.2,19.05
  pour Top (no thermals): 108.58,13.97 111.12,13.97 111.12,12.7 109.86,11.43 106.93,11.43 106.93,12.32
N$31
  Top 0.635: L3.2 10.35,45.51 U7.1
  Top 1.27: L3.2 9.39,52.07 D12.A
N$32
  Bottom 0.305: JMP2.2 19.3,48.64 R26.E
N$33
  Top 0.305: U7.3 14.73,44.11 16.59,45.97 R26.S
N$34  (via drill 0.35)
  Top 0.305: C12.1 7.87,50.27 8.13,50.01 v8.13,49.28 | v13.97,48.01 12.7,46.74 U7.5
  Top 0.635: JP1.1 3.28,50.27 3.81,50.27 | 3.81,50.27 C12.1 | D12.C 3.56,50.52 3.81,50.27
  Top 1.27: D12.C 3.56,50.55 | JP1.1 3.56,50.55 | 3.56,50.55 5.81,50.55 C12.1
  Bottom 0.305: v13.97,48.01 8.89,48.01 8.13,48.77 v8.13,49.28
N$35  (via drill 0.35)
  Top 0.305: R25.2 9.08,43.75 v10.92,41.91
  Top 1.27: JP1.2 3.47,46.57 R24.1 3.47,42.93 4.04,42.35 6.76,42.35 8.13,43.72 R25.2
  Bottom 0.305: v10.92,41.91 15.75,41.91 15.75,43.18 16,43.43 R26.A
N$41
  Top 0.635: D14.A 8.25,37.34 | L5.2 10.35,29 U9.1
  Top 1.27: 8.25,37.34 10.03,35.56 L5.2
N$42
  Bottom 0.305: JMP4.2 19.3,32.13 R32.E
N$43
  Top 0.305: U9.3 14.73,27.6 16.59,29.46 R32.S
N$44  (via drill 0.35)
  Top 0.305: C16.1 7.87,33.76 8.13,33.5 v8.13,32.77 | v13.97,31.5 12.7,30.23 U9.5
  Top 0.635: 3.28,33.76 3.81,33.76 | 3.81,33.76 C16.1 | D14.C 3.56,34.01 3.81,33.76
  Top 1.27: D14.C 3.56,34.04 JP2.1 3.28,33.76 C16.1
  Bottom 0.305: v13.97,31.5 8.89,31.5 8.13,32.26 v8.13,32.77
N$45  (via drill 0.35)
  Top 0.305: R31.2 9.08,27.24 v10.92,25.4
  Top 1.27: JP2.2 3.47,30.06 R30.1 3.47,26.09 7.01,26.09 8.13,27.21 R31.2
  Bottom 0.305: v10.92,25.4 15.75,25.4 15.75,26.67 16,26.92 R32.A
N$51
  Top 0.635: D16.A 4.57,8.57 L7.2 6.98,10.35 12.91,10.35 U11.1
  Top 1.27: D16.A 4.57,7.94 6.98,10.35
N$52
  Bottom 0.305: JMP6.2 9.78,19.3 R38.E
N$53
  Top 0.305: U11.3 14.31,14.73 12.45,16.59 R38.S
N$54  (via drill 0.35)
  Top 0.305: C20.1 8.15,7.87 8.41,8.13 v9.14,8.13 | v10.41,13.97 11.68,12.7 U11.5
  Top 0.635: 8.15,3.28 8.15,3.81 | 8.15,3.81 C20.1 | D16.C 7.91,3.56 8.15,3.81
  Top 1.27: D16.C 7.87,3.56 JP3.1 8.15,3.28 C20.1
  Bottom 0.305: v10.41,13.97 10.41,8.89 9.65,8.13 v9.14,8.13
N$55  (via drill 0.35)
  Top 0.305: R37.2 14.67,9.08 v16.51,10.92
  Top 0.635: 11.85,3.47 R36.1 14.48,3.47
  Top 1.27: JP3.2 11.85,3.47 14.48,3.47 | R36.1 15.94,3.47 15.94,6.86 R37.2
  Bottom 0.305: v16.51,10.92 16.51,15.75 15.24,15.75 14.99,16 R38.A
N$61
  Top 0.635: L9.2 29.42,10.35 U13.1
  Top 1.27: D18.A 21.08,8.57 L9.2
N$62
  Bottom 0.305: JMP8.2 26.29,19.3 R44.E
N$63
  Top 0.305: U13.3 30.82,14.73 28.96,16.59 R44.S
N$64  (via drill 0.35)
  Top 0.305: C24.1 24.66,6.35 24.66,7.87 24.92,8.13 v25.65,8.13 | v26.92,13.97 28.19,12.7 U13.5
  Top 0.635: 24.66,3.28 24.66,3.81 | 24.66,3.81 C24.1 | 24.42,3.56 24.66,3.81
  Top 1.27: JP4.1 24.66,3.28 24.66,6.35 | D18.C 24.42,3.56
  Bottom 0.305: v26.92,13.97 26.92,8.89 26.16,8.13 v25.65,8.13
N$65  (via drill 0.35)
  Top 0.305: R43.2 31.18,9.08 v33.02,10.92
  Top 1.27: JP4.2 28.36,3.47 R42.1 33.34,3.47 33.34,5.99 31.21,8.13 R43.2
  Bottom 0.305: v33.02,10.92 33.02,15.75 31.75,15.75 31.5,16 R44.A
RF_INT  (via drill 0.35)
  Top 0.305: v59.69,17.78 60.96,16.51 63.5,16.51 M1.8 | v59.69,43.18 v67.31,43.18
  Bottom 0.305: v59.69,17.78 v59.69,43.18 | v67.31,43.18 78.74,43.18 79.38,43.81 U2.P$13
RIGHT_BTN  (via drill 0.35)
  Top 0.406: v107.31,35.56 102.23,40.64 U2.P$4
  Bottom 0.406: v107.31,35.56 J3.5
RIGHT_CTRL  (via drill 0.35)
  Top 0.254: U13.4 28.62,15.2 v27.94,15.88 | v27.94,25.4 31.8,29.26 v33.66,29.26 | v57.15,40.01 59.05,41.91 67.44,41.91 68.44,42.92 R27.1 | v45.08,29.21 v57.15,29.21
  Top 0.305: R27.1 U2.P$17
  Bottom 0.254: v27.94,15.88 v27.94,25.4 | v33.66,29.26 45.04,29.26 v45.08,29.21 | v57.15,29.21 v57.15,40.01
TAIL_BTN  (via drill 0.35)
  Top 0.406: v108.58,40.64 107.31,41.91 U2.P$2
  Bottom 0.406: v108.58,40.64 J3.3
TAIL_CTRL  (via drill 0.35)
  Top 0.254: U9.4 14.58,30.73 25.5,30.73 v25.52,30.75 | v58.59,30.86 58.46,30.73 v45.21,30.73 | v58.46,38.73 60.37,40.64 71.75,40.64 74.03,42.92 R22.1
  Top 0.305: R22.1 U2.P$15
  Bottom 0.254: v25.52,30.75 25.75,30.75 26.4,31.4 30.76,31.4 32.44,33.08 42.87,33.08 v45.21,30.73 | v58.46,38.73 58.59,38.61 v58.59,30.86
V+  (via drill 0.35, 1)
  Top 0.305: U13.6 24.57,11.75 23.62,12.7 23.62,14.29 L9.1 | U11.6 8.06,11.75 7.11,12.7 7.11,14.29 L7.1 6.06,15.05 | U9.6 11.75,33.85 12.7,34.8 14.29,34.8 L5.1 | U7.6 11.75,50.36 12.7,51.31 14.29,51.31 L3.1 | U5.5 107.09,16.58 G2.4 | LED3.A 69,2.63 v69.09,2.54 | R6.2 80.85,20.67 86.96,14.57 J5.1
  Top 0.406: TP2.TP 23.24,32.89 v21.08,35.05
  Top 0.635: 22.57,15.05 L9.1 | v20.34,21.08 v23.37,21.08 | v3.83,21.08 v6.86,21.08 | 18.42,38.08 C15.1 21.08,38.08 v21.08,35.05 | C11.1 21.08,54.59 v21.08,51.56
  Top 1.27: 22.57,15.05 20.34,17.27 C23.1 v20.34,21.08 21.59,22.33 v21.59,22.86 | 6.06,15.05 3.83,17.27 C19.1 v3.83,21.08 2.41,21.08 v1.91,21.59 | L5.1 17.57,38.08 18.42,38.08 | L3.1 17.57,54.59 C11.1 20.34,55.88 v20.95,55.88 v22.22,55.88 | C15.1 20.34,39.37 v20.95,39.37 v22.22,39.37 | C8.1 42.84,28.07
  Top 2.54: R28.E 109.22,25.4 v105.41,25.4 v102.87,25.4 v100.33,25.4 v97.79,25.4 v95.25,25.4 | v95.25,25.4 86.96,17.11 86.96,14.57 | v95.25,25.4 69.85,25.4 68.58,26.67 44.24,26.67 42.84,28.07
  Bottom 0.305: v69.09,2.54 70.36,3.81 74.93,3.81 76.71,2.03 80.9,2.03 83.19,4.32 83.19,11.43 86.28,14.53 J5.1 | 23.5,26.67 23.5,24.77 v21.59,22.86
  Bottom 3.81: J5.1 83.89,11.43 41.91,11.43 38.1,15.24 38.1,20.95 31.11,27.94 24.77,27.94 23.5,26.67
  pour Top (no thermals): 111.12,27.94 111.12,22.86 109.86,21.59 109.86,14.86 106.17,14.86 106.17,24.13 94.61,24.13 93.34,25.4 95.88,27.94
  pour Bottom (no thermals): 84.45,12.7 89.53,12.7 89.53,17.78 95.25,23.5 110.62,23.5 110.62,27.3 94.61,27.3 84.45,17.14
  pour Bottom (no thermals): 0.64,20.32 0.64,21.59 3.17,24.13 18.42,24.13 19.69,25.4 19.69,55.88 20.95,57.15 23.5,57.15 24.77,55.88 24.77,21.59 23.5,20.32
  pour Top (no thermals): 41.4,25.4 43.81,25.4 43.81,30.48 43.18,31.11 41.4,31.11
VCC
  Top 0.406: J1.2 107.31,2.54 106.05,1.27 80.64,1.27 79.38,2.54 D10.C
  pour Top (no thermals): 104.78,12.19 106.3,12.19 106.3,8.64 106.68,8.26 107.95,8.26 108.58,7.62 108.58,2.54 107.95,1.91 106.68,1.91 104.78,3.81

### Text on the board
tValues: GND | ENC | 5V | 3V3 | RPI ON SERIAL1 | GND | HEAD | 3V3 | TAIL | GPS ON SERIAL2 | LEFT | 5V | RIGHT | V+ | GND | GND | PA4-CS / PA1-EN / PB5-INT
bValues: HEAD+ | RPI ON SERIAL1 | GND | ENC | 5V | 3V3 | GND | HEAD | 3V3 | TAIL | GPS ON SERIAL2 | CAD | LEFT | 5V | GND | ANA.BAT. | GND | RIGHT | TAIL+ | GND | Above here lies / the 5V regulator | PA4-CS / PA1-EN / PB5-INT | Above here are / protection circuits / for reverse polarity, / over/under-voltage | University of Toronto Human Powered Vehicle Design Team / Blueshift Digital Electronics Board V.3 / hpv@hpvdt.skule.ca | GND | +BAT | LEFT+ | RIGHT+

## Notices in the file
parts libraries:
diy-modules: Released under the Creative Commons Attribution 4.0 International License: http://creativecommons.org/licenses/by/4.0
